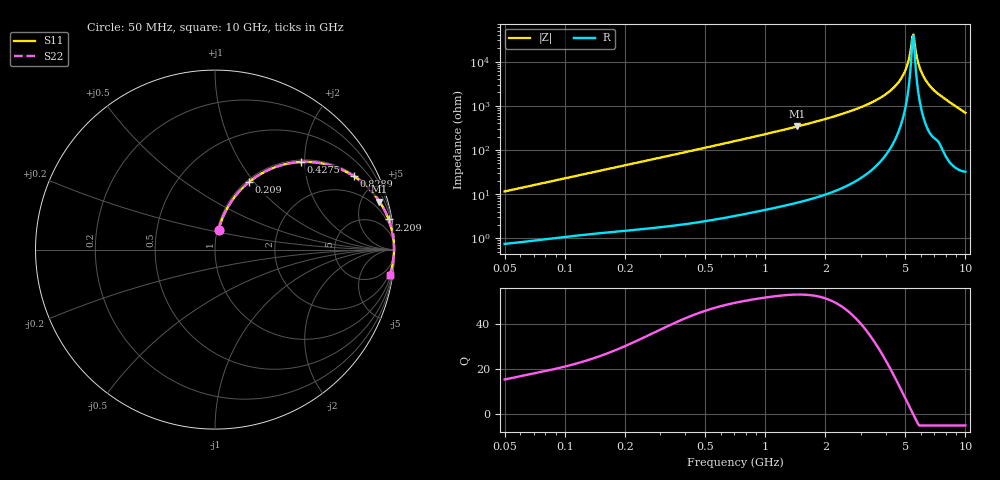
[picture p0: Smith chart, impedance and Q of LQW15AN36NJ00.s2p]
!Murata Part Number: LQW15AN36NJ00
!These Parameters are Measured in Series Mode Connection
!  o--[Z]--o
!Port1  Port2
!  o-------o
!Freq. Start=50[MHz] Stop=10[GHz], 401[Steps]
# Hz S RI R 50
!Freq.(Hz)	S 11(Real)	S 11(Imag)	S 21(Real)	S 21(Imag)	S 12(Real)	S 12(Imag)	S 22(Real)	S 22(Imag)
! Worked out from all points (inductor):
!   401 points, 50 MHz to 10 GHz, reference 50 ohm
!   read as one part in series: L = 36.4 nH near 51.34 MHz
!   highest Q = 53 at 1.446 GHz (marker M1), where L = 37.4 nH
!   self-resonance near 5.437 GHz
!   S11 on the Smith chart (normalised r, x): 50 MHz: 1.01, +0.23; 209 MHz: 1.03, +0.94; 427.5 MHz: 1.04, +1.91; 828.9 MHz: 1.07, +3.74; 2.209 GHz: 1, +11; 10 GHz: 2, -14
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5e7  0.0202 0.1118  0.9798 -0.1118  0.9798 -0.1118  0.0202 0.1118
1.214486e8  0.0793 0.2495  0.9207 -0.2495  0.9207 -0.2495  0.0793 0.2495
2.09049e8  0.1875 0.3745  0.8125 -0.3745  0.8125 -0.3745  0.1875 0.3745
2.949953e8  0.3073 0.4481  0.6927 -0.4481  0.6927 -0.4481  0.3073 0.4481
4.274518e8  0.477 0.4881  0.523 -0.4881  0.523 -0.4881  0.477 0.4881
7.071068e8  0.7119 0.4428  0.2881 -0.4428  0.2881 -0.4428  0.7119 0.4428
8.289263e8  0.773 0.4091  0.227 -0.4091  0.227 -0.4091  0.773 0.4091
1.445853e9  0.9161 0.268  0.0839 -0.268  0.0839 -0.268  0.9161 0.268
1.717543e9  0.9414 0.2255  0.0586 -0.2255  0.0586 -0.2255  0.9414 0.2255
2.209055e9  0.9672 0.1683  0.0328 -0.1683  0.0328 -0.1683  0.9672 0.1683
3.243629e9  0.9889 0.092  0.0111 -0.092  0.0111 -0.092  0.9889 0.092
4.171863e9  0.9955 0.0473  0.00451 -0.0473  0.00451 -0.0473  0.9955 0.0473
4.890587e9  0.9974 0.0199  0.00261 -0.0199  0.00261 -0.0199  0.9974 0.0199
5.156693e9  0.9977 0.0107  0.00235 -0.0107  0.00235 -0.0107  0.9977 0.0107
5.365732e9  0.9977 0.0038  0.00227 -0.0038  0.00227 -0.0038  0.9977 0.0038
5.509778e9  0.9977 -0.000844  0.00228 0.000844  0.00228 0.000844  0.9977 -0.000844
5.583245e9  0.9977 -0.00318  0.00231 0.00318  0.00231 0.00318  0.9977 -0.00318
5.809576e9  0.9975 -0.0102  0.00246 0.0102  0.00246 0.0102  0.9975 -0.0102
5.965537e9  0.9974 -0.015  0.00265 0.015  0.00265 0.015  0.9974 -0.015
6.54512e9  0.9961 -0.0322  0.00393 0.0322  0.00393 0.0322  0.9961 -0.0322
7.37379e9  0.9926 -0.0544  0.00744 0.0544  0.00744 0.0544  0.9926 -0.0544
1e10  0.9733 -0.1396  0.0267 0.1396  0.0267 0.1396  0.9733 -0.1396
